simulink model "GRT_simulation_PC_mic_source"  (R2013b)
settings: Solver=FixedStepDiscrete  SolverMode=MultiTasking  StartTime=0.0  StopTime=inf  FixedStep=1/Param.Fs  RelTol=1e-3
InitFcn:
  | clear all; clc; close all;
  | Param  = Config_parameter();
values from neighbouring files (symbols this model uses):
  FFTLen = 2^(ceil(log(nFrmLen)/log(2)))    [DFT_FilterBank_Analysis_func.m]    (also in DFT_FilterBank_Synthesis_func.m; main_run3.m)
  nHopSize = size(in_frame_seg,1)    [DFT_FilterBank_Analysis_func.m]    (also in DFT_FilterBank_Synthesis_func.m = size(ref_out,1); main_run3.m = 16)
  nNumChs = size(ref_out,1)    [DFT_FilterBank_Analysis_func.m]    (also in DFT_FilterBank_Synthesis_func.m = size(in_frame,2); main_run3.m = 32; OLA_func.m = size(in_frame,2); PDbranchingsmooth_sm.m = size(x,1))
undefined symbols (not defined in the file or in its folder): a_dd, AFC_switch, DownSample_factor, DownSamplingFactor, eta, Freq_shift, Fs, mu, prototype_win, VarAmpSwitch, VarAttackTime, VarCompressRatio, VarCompressTh, VarFs, VarKneeWidth, VarLimiterCompressRatio, VarLimiterTh, VarMaxSPL, VarMicNoiseCompressRatio, VarMicNoiseTh, VarRefGaindB, VarRefSPL, VarReleaseTime, VarSwitch, VarThdB, Wiener_switch
libraries: dspadpt3 x1, dspbuff3 x1, dspsrcs4 x1, dspsnks4 x1

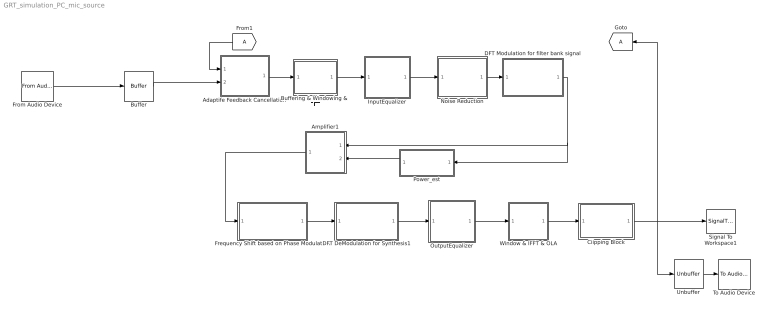
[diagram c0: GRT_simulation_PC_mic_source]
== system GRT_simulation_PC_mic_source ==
  Adaptife Feedback Cancellation : Subsystem
  Amplifier1 : Subsystem
  Buffer : Buffer  N=Param.IO_FrameSize  TreatMby1Signals=One channel
  Buffering & Windowing &  FFT : Subsystem
  Ciipping Block : Subsystem
  DFT DeModulation for Synthesis1 : Subsystem
  DFT Modulation for filter bank signal : Subsystem
  Frequency Shift based on Phase Modulation : Subsystem
  From Audio Device : dspsrcs4/From Audio Device  deviceName=Microphone (Realtek High Definition Audio)  numChannels=1  sampleRate=Param.Fs  deviceDatatype=Determine from output data type  autoBufferSize=on  bufferSize=160  queueDuration=1/Param.Fs  frameSize=1  outputDatatype=double  defaultInputChannelMapping=on  inputChannelMapping=1:2
  From1 : From
  Goto : Goto
  InputEqualizer : MATLAB Function  TreatAsAtomicUnit=on
  Noise Reduction : Subsystem
  OutputEqualizer : MATLAB Function  TreatAsAtomicUnit=on
  Power_est : Subsystem
  Signal To Workspace1 : SignalToWorkspace  Commented=on  VariableName=yout1
  To Audio Device : dspsnks4/To Audio Device  deviceName=Speakers (Realtek High Definition Audio)  inheritSampleRate=on  sampleRate=44100  deviceDatatype=Determine from input data type  autoBufferSize=on  bufferSize=160  queueDuration=1/Param.Fs  defaultOutputChannelMapping=on  outputChannelMapping=1:2
  Unbuffer : Unbuffer  SampleBasedProcessing=Same as frame based
  Window & IFFT & OLA : Subsystem
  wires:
  Window & IFFT & OLA/1(Out1) -> Ciipping Block/1(In1)
  DFT DeModulation for Synthesis1/1(Out1) -> OutputEqualizer/1(InFreq)
  Frequency Shift based on Phase Modulation/1(Out1) -> DFT DeModulation for Synthesis1/1(In1)
  DFT Modulation for filter bank signal/1(Out1) -> Amplifier1/1(In1), Power_est/1(In1)
  Amplifier1/1(Out1) -> Frequency Shift based on Phase Modulation/1(In1)
  Noise Reduction/1(Out1) -> DFT Modulation for filter bank signal/1(In1)
  Buffering & Windowing &  FFT/1(Out1) -> InputEqualizer/1(InFreq)
  From1/1 -> Adaptife Feedback Cancellation/1(In1)
  Buffer/1 -> Adaptife Feedback Cancellation/2(In2)
  Adaptife Feedback Cancellation/1(Out1) -> Buffering & Windowing &  FFT/1(In1)
  From Audio Device/1 -> Buffer/1
  InputEqualizer/1(OutFreqCal) -> Noise Reduction/1(In1)
  OutputEqualizer/1(OutFreqCal) -> Window & IFFT & OLA/1(In1)
  Ciipping Block/1(Out1) -> Unbuffer/1, Goto/1, Signal To Workspace1/1
  Power_est/1(Out1) -> Amplifier1/2(In2)
  Unbuffer/1 -> To Audio Device/1

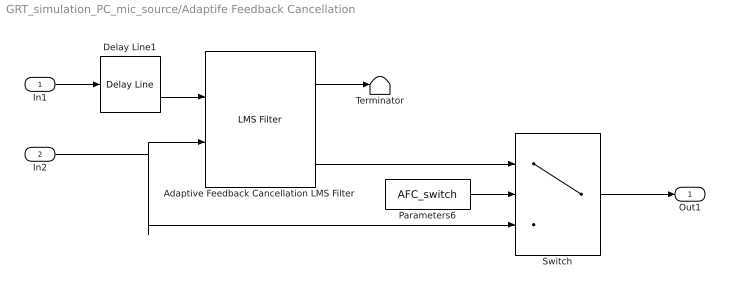
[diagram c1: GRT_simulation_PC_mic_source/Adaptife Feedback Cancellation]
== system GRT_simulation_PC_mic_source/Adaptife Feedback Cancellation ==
  In1 : Inport
  In2 : Inport  Port=2
  Adaptive Feedback Cancellation LMS Filter : dspadpt3/LMS Filter  Algo=LMS  L=128  stepflag=Dialog  mu=0.002  leakage=1.0  ic=0  Adapt=off  resetflag=None  weights=off  secondCoeffMode=User-defined  secondCoeffWordLength=2  secondCoeffFracLength=15  accum2Mode=User-defined  accum2FracLength=20  prodOutput2Mode=User-defined  prodOutput2FracLength=20  prodOutput3Mode=User-defined  prodOutput3FracLength=20  prodOutput4Mode=User-defined  prodOutput4FracLength=20  quotientMode=User-defined  quotientFracLength=20  roundingMode=Floor  overflowMode=off  addnparflag=off
  Delay Line1 : dspbuff3/Delay Line  siz=Param.IO_FrameSize  ic=0  directfeed=off  enable_output=off  hold_output=off  TreatMby1Signals=One channel
  Parameters6 : Constant  Value=AFC_switch
  Switch : Switch  Criteria=u2 > Threshold
  Terminator : Terminator
  Out1 : Outport
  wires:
  Parameters6/1 -> Switch/2
  Switch/1 -> Out1/1
  Delay Line1/1 -> Adaptive Feedback Cancellation LMS Filter/1
  Adaptive Feedback Cancellation LMS Filter/1 -> Terminator/1
  Adaptive Feedback Cancellation LMS Filter/2 -> Switch/1
  In1/1 -> Delay Line1/1
  In2/1 -> Switch/3, Adaptive Feedback Cancellation LMS Filter/2

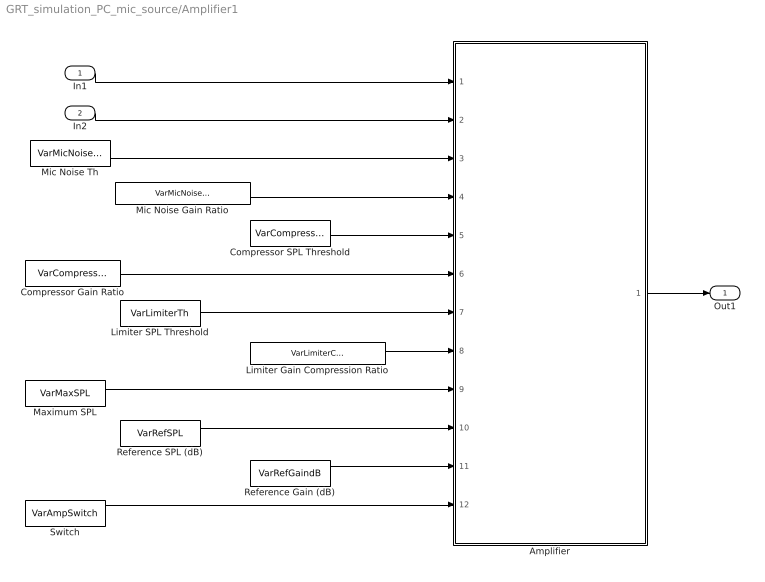
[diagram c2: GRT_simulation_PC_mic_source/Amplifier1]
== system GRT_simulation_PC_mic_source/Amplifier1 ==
  In1 : Inport
  In2 : Inport  Port=2
  Amplifier : MATLAB Function  TreatAsAtomicUnit=on
  Compressor Gain Ratio : Constant  Value=VarCompressRatio  VectorParams1D=off
  Compressor SPL Threshold : Constant  Value=VarCompressTh  VectorParams1D=off
  Limiter Gain Compression Ratio : Constant  Value=VarLimiterCompressRatio  VectorParams1D=off
  Limiter SPL Threshold : Constant  Value=VarLimiterTh  VectorParams1D=off
  Maximum SPL : Constant  Value=VarMaxSPL  VectorParams1D=off
  Mic Noise Gain Ratio : Constant  Value=VarMicNoiseCompressRatio  VectorParams1D=off
  Mic Noise Th : Constant  Value=VarMicNoiseTh  VectorParams1D=off
  Reference Gain (dB) : Constant  Value=VarRefGaindB  VectorParams1D=off
  Reference SPL (dB) : Constant  Value=VarRefSPL  VectorParams1D=off
  Switch : Constant  Value=VarAmpSwitch  VectorParams1D=off
  Out1 : Outport
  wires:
  In1/1 -> Amplifier/1(in_FBSig)
  Amplifier/1(Out_FBSig) -> Out1/1
  In2/1 -> Amplifier/2(in_EstdB)
  Compressor SPL Threshold/1 -> Amplifier/5(CT)
  Mic Noise Gain Ratio/1 -> Amplifier/4(ER)
  Mic Noise Th/1 -> Amplifier/3(ET)
  Reference Gain (dB)/1 -> Amplifier/11(G0)
  Reference SPL (dB)/1 -> Amplifier/10(L0)
  Maximum SPL/1 -> Amplifier/9(Lmax)
  Limiter Gain Compression Ratio/1 -> Amplifier/8(LR)
  Limiter SPL Threshold/1 -> Amplifier/7(LT)
  Compressor Gain Ratio/1 -> Amplifier/6(CR)
  Switch/1 -> Amplifier/12(AmpSwitch)

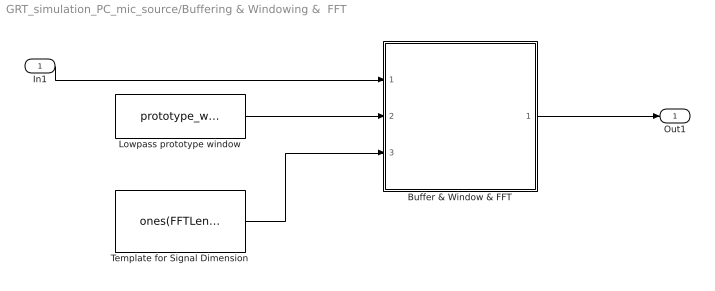
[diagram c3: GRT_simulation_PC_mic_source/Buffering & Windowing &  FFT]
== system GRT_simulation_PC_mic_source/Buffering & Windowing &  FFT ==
  In1 : Inport
  Buffer & Window & FFT : MATLAB Function  TreatAsAtomicUnit=on
  Lowpass prototype window : Constant  Value=prototype_win  VectorParams1D=off
  Template for Signal Dimension : Constant  Value=ones(FFTLen,nNumChs)  VectorParams1D=off
  Out1 : Outport
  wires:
  In1/1 -> Buffer & Window & FFT/1(in_frame_seg)
  Buffer & Window & FFT/1(FreqOut) -> Out1/1
  Template for Signal Dimension/1 -> Buffer & Window & FFT/3(ref_out)
  Lowpass prototype window/1 -> Buffer & Window & FFT/2(win)

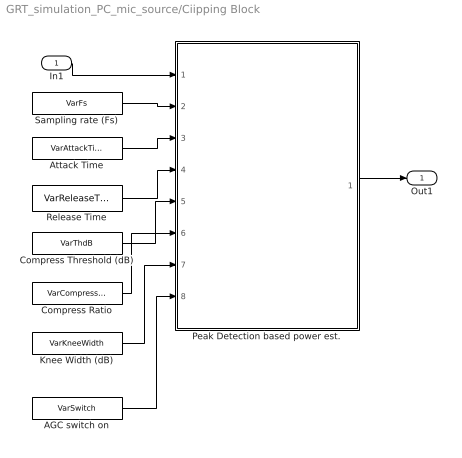
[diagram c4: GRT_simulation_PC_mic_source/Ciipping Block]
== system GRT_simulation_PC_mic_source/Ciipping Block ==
  In1 : Inport
  AGC switch on : Constant  Value=VarSwitch  VectorParams1D=off
  Attack Time : Constant  Value=VarAttackTime  VectorParams1D=off
  Compress Ratio : Constant  Value=VarCompressRatio  VectorParams1D=off
  Compress Threshold (dB) : Constant  Value=VarThdB  VectorParams1D=off
  Knee Width (dB) : Constant  Value=VarKneeWidth  VectorParams1D=off
  Peak Detection based power est. : MATLAB Function  TreatAsAtomicUnit=on
  Release Time : Constant  Value=VarReleaseTime  VectorParams1D=off
  Sampling rate (Fs) : Constant  Value=VarFs  VectorParams1D=off
  Out1 : Outport
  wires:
  In1/1 -> Peak Detection based power est./1(x)
  Peak Detection based power est./1(y) -> Out1/1
  Sampling rate (Fs)/1 -> Peak Detection based power est./2(fs)
  Attack Time/1 -> Peak Detection based power est./3(tauAttack)
  Release Time/1 -> Peak Detection based power est./4(tauRelease)
  Compress Threshold (dB)/1 -> Peak Detection based power est./5(Threshold)
  Knee Width (dB)/1 -> Peak Detection based power est./7(KneeWidth)
  Compress Ratio/1 -> Peak Detection based power est./6(ratio)
  AGC switch on/1 -> Peak Detection based power est./8(AGCSwitch)

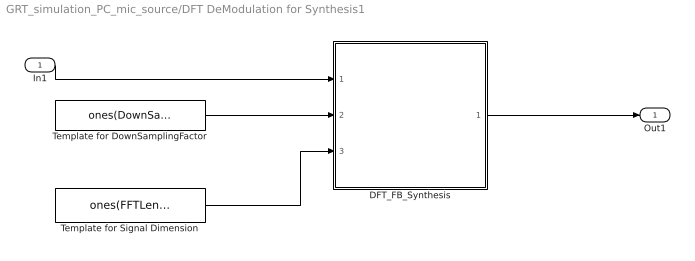
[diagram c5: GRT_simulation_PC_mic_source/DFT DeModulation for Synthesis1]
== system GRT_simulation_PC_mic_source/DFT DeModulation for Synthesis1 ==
  In1 : Inport
  DFT_FB_Synthesis : MATLAB Function  TreatAsAtomicUnit=on
  Template for DownSamplingFactor : Constant  Value=ones(DownSample_factor,1)  VectorParams1D=off
  Template for Signal Dimension : Constant  Value=ones(FFTLen,nHopSize)  VectorParams1D=off
  Out1 : Outport
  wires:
  In1/1 -> DFT_FB_Synthesis/1(FB_In)
  DFT_FB_Synthesis/1(Out_FFTSig) -> Out1/1
  Template for DownSamplingFactor/1 -> DFT_FB_Synthesis/2(ref_DownSample_factor)
  Template for Signal Dimension/1 -> DFT_FB_Synthesis/3(ref_out)

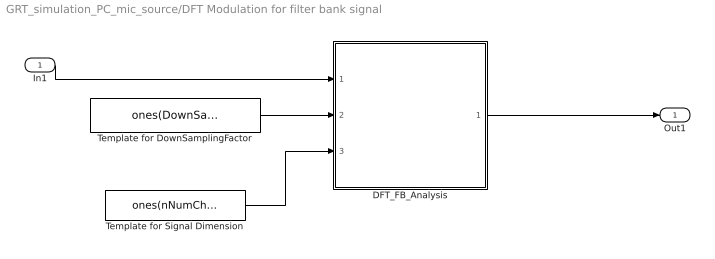
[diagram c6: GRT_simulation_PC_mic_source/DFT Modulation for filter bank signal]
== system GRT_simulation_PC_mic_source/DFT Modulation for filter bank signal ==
  In1 : Inport
  DFT_FB_Analysis : MATLAB Function  TreatAsAtomicUnit=on
  Template for DownSamplingFactor : Constant  Value=ones(DownSample_factor,1)  VectorParams1D=off
  Template for Signal Dimension : Constant  Value=ones(nNumChs,nHopSize)  VectorParams1D=off
  Out1 : Outport
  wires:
  Template for DownSamplingFactor/1 -> DFT_FB_Analysis/2(ref_DownSample_factor)
  Template for Signal Dimension/1 -> DFT_FB_Analysis/3(ref_out)
  DFT_FB_Analysis/1(FB_Out) -> Out1/1
  In1/1 -> DFT_FB_Analysis/1(in_FFTSig)

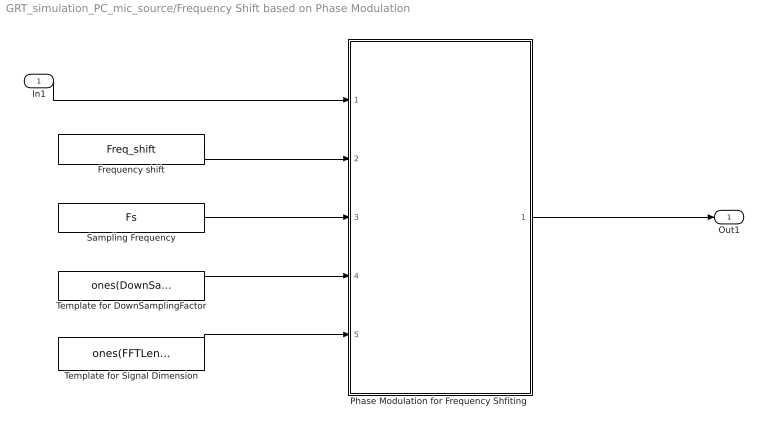
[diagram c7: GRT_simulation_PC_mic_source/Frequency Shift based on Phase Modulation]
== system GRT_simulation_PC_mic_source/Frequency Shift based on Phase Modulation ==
  In1 : Inport
  Frequency shift : Constant  Value=Freq_shift  VectorParams1D=off
  "Phase Modulation for Frequency Shfiting " : MATLAB Function  TreatAsAtomicUnit=on
  Sampling Frequency : Constant  Value=Fs  VectorParams1D=off
  Template for DownSamplingFactor : Constant  Value=ones(DownSample_factor,1)  VectorParams1D=off
  Template for Signal Dimension : Constant  Value=ones(FFTLen,nHopSize)  VectorParams1D=off
  Out1 : Outport
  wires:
  In1/1 -> "Phase Modulation for Frequency Shfiting "/1(FB_In)
  "Phase Modulation for Frequency Shfiting "/1(FreqShiftOut) -> Out1/1
  Template for DownSamplingFactor/1 -> "Phase Modulation for Frequency Shfiting "/4(ref_Downsample_factor)
  Template for Signal Dimension/1 -> "Phase Modulation for Frequency Shfiting "/5(ref_out)
  Frequency shift/1 -> "Phase Modulation for Frequency Shfiting "/2(Pm_freq)
  Sampling Frequency/1 -> "Phase Modulation for Frequency Shfiting "/3(Fs)

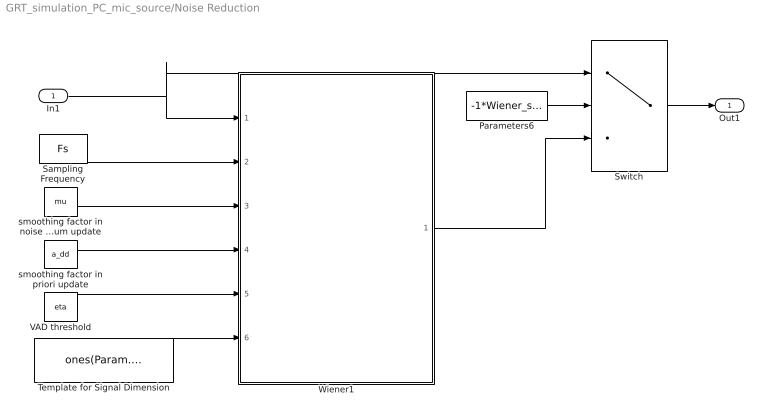
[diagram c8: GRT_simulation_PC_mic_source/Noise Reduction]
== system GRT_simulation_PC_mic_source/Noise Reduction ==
  In1 : Inport
  Parameters6 : Constant  Value=-1*Wiener_switch
  Sampling Frequency : Constant  Value=Fs  VectorParams1D=off
  Switch : Switch
  Template for Signal Dimension : Constant  Value=ones(Param.IO_FrameSize,1)  VectorParams1D=off
  VAD threshold : Constant  Value=eta  VectorParams1D=off
  Wiener1 : MATLAB Function  TreatAsAtomicUnit=on
  smoothing factor in noise spectrum update : Constant  Value=mu  VectorParams1D=off
  smoothing factor in priori update : Constant  Value=a_dd  VectorParams1D=off
  Out1 : Outport
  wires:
  In1/1 -> Switch/1, Wiener1/1(NoisyFreq)
  Sampling Frequency/1 -> Wiener1/2(Fs)
  Wiener1/1(EnhanFreq) -> Switch/3
  smoothing factor in noise spectrum update/1 -> Wiener1/3(mu)
  smoothing factor in priori update/1 -> Wiener1/4(a_dd)
  VAD threshold/1 -> Wiener1/5(eta)
  Template for Signal Dimension/1 -> Wiener1/6(ref_out)
  Switch/1 -> Out1/1
  Parameters6/1 -> Switch/2

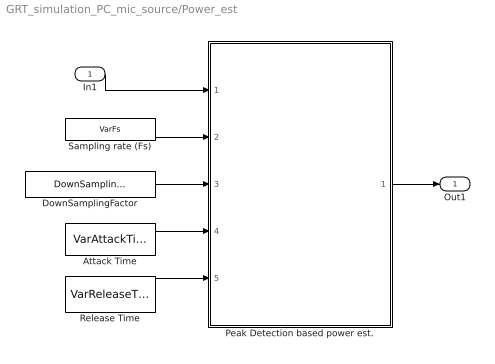
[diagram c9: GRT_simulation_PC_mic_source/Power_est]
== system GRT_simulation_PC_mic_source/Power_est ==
  In1 : Inport
  Attack Time : Constant  Value=VarAttackTime  VectorParams1D=off
  DownSamplingFactor : Constant  Value=DownSamplingFactor  VectorParams1D=off
  Peak Detection based power est. : MATLAB Function  TreatAsAtomicUnit=on
  Release Time : Constant  Value=VarReleaseTime  VectorParams1D=off
  Sampling rate (Fs) : Constant  Value=VarFs  VectorParams1D=off
  Out1 : Outport
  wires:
  In1/1 -> Peak Detection based power est./1(x)
  Peak Detection based power est./1(lg) -> Out1/1
  Sampling rate (Fs)/1 -> Peak Detection based power est./2(fs)
  Attack Time/1 -> Peak Detection based power est./4(tauAttack)
  Release Time/1 -> Peak Detection based power est./5(tauRelease)
  DownSamplingFactor/1 -> Peak Detection based power est./3(DownSamplingFactor)

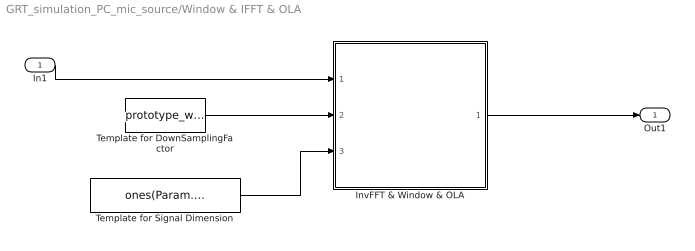
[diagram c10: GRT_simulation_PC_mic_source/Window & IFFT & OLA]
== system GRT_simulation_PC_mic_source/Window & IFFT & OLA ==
  In1 : Inport
  InvFFT & Window & OLA : MATLAB Function  TreatAsAtomicUnit=on
  Template for DownSamplingFactor : Constant  Value=prototype_win  VectorParams1D=off
  Template for Signal Dimension : Constant  Value=ones(Param.IO_FrameSize,1)  VectorParams1D=off
  Out1 : Outport
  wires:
  Template for Signal Dimension/1 -> InvFFT & Window & OLA/3(ref_out)
  Template for DownSamplingFactor/1 -> InvFFT & Window & OLA/2(win)
  InvFFT & Window & OLA/1(TimeSegOut) -> Out1/1
  In1/1 -> InvFFT & Window & OLA/1(FreqIn)
